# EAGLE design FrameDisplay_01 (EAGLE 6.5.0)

## Sheet 1 of 2: DISPLAY
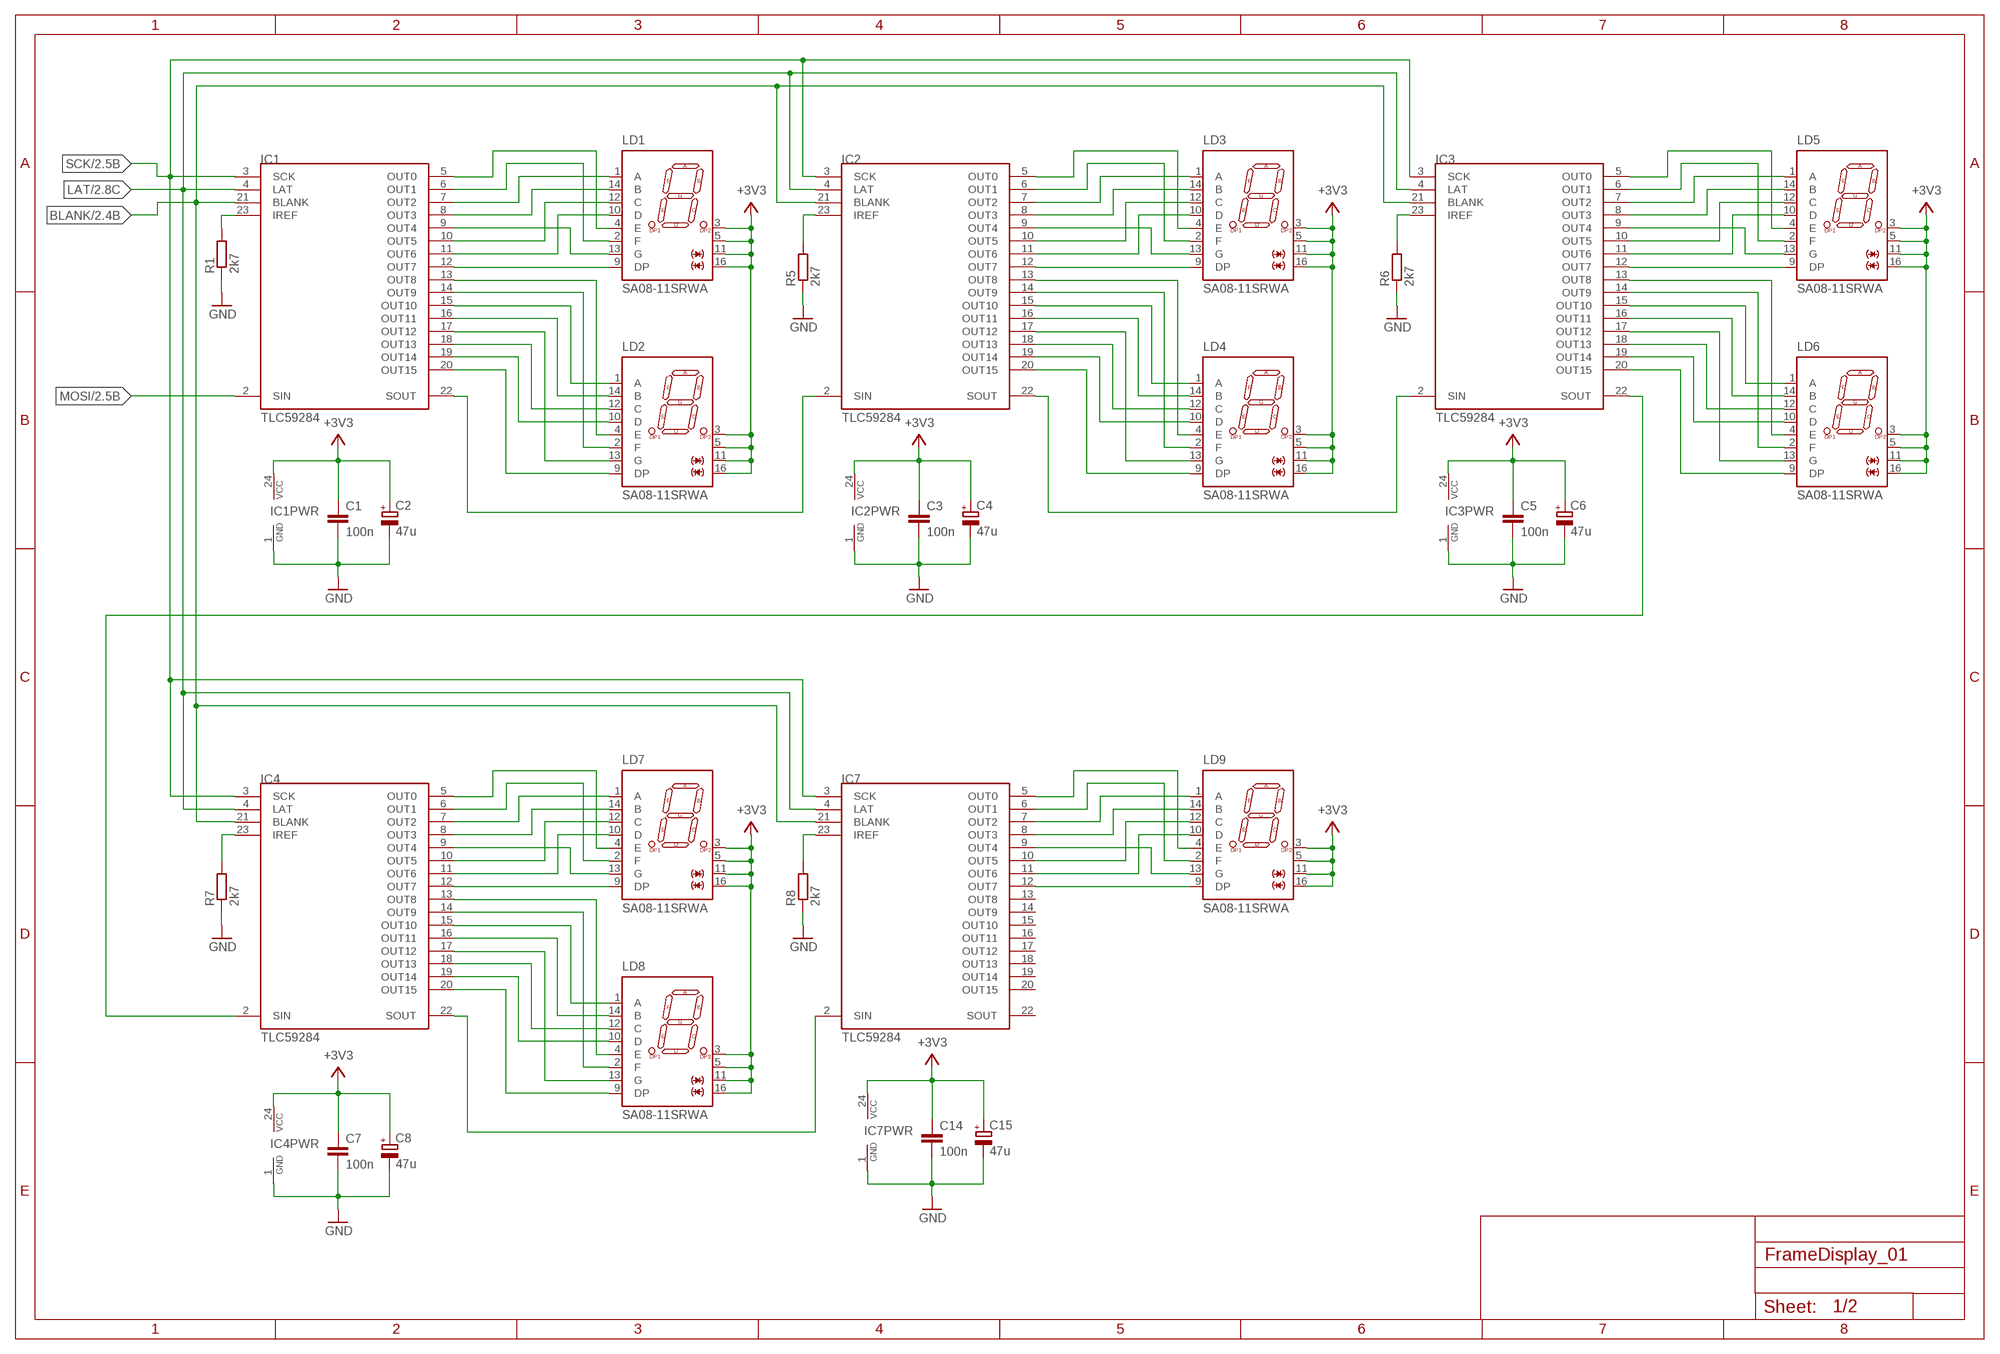
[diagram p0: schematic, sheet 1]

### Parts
C1  100n  C-EUC0603  [C0603]
C2  47u  CPOL-EUCT3216  [CT3216]
C3  100n  C-EUC0603  [C0603]
C4  47u  CPOL-EUCT3216  [CT3216]
C5  100n  C-EUC0603  [C0603]
C6  47u  CPOL-EUCT3216  [CT3216]
C7  100n  C-EUC0603  [C0603]
C8  47u  CPOL-EUCT3216  [CT3216]
C14  100n  C-EUC0603  [C0603]
C15  47u  CPOL-EUCT3216  [CT3216]
IC1  TLC59284  [SSOP24-25MIL]
IC2  TLC59284  [SSOP24-25MIL]
IC3  TLC59284  [SSOP24-25MIL]
IC4  TLC59284  [SSOP24-25MIL]
IC7  TLC59284  [SSOP24-25MIL]
LD1  SA08-11SRWA  SA08-11  [SA08]
LD2  SA08-11SRWA  SA08-11  [SA08]
LD3  SA08-11SRWA  SA08-11  [SA08]
LD4  SA08-11SRWA  SA08-11  [SA08]
LD5  SA08-11SRWA  SA08-11  [SA08]
LD6  SA08-11SRWA  SA08-11  [SA08]
LD7  SA08-11SRWA  SA08-11  [SA08]
LD8  SA08-11SRWA  SA08-11  [SA08]
LD9  SA08-11SRWA  SA08-11  [SA08]
R1  2k7  R-EU_R0603  [R0603]
R5  2k7  R-EU_R0603  [R0603]
R6  2k7  R-EU_R0603  [R0603]
R7  2k7  R-EU_R0603  [R0603]
R8  2k7  R-EU_R0603  [R0603]

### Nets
+3V3: C1.1 C2.+ C3.1 C4.+ C5.1 C6.+ C7.1 C8.+ C14.1 C15.+ IC1.24(PWR:VCC) IC2.24(PWR:VCC) IC3.24(PWR:VCC) IC4.24(PWR:VCC) IC7.24(PWR:VCC) LD1.3(AK) LD1.5(AK) LD1.11(AK) LD1.16(AK) LD2.3(AK) LD2.5(AK) LD2.11(AK) LD2.16(AK) LD3.3(AK) LD3.5(AK) LD3.11(AK) LD3.16(AK) LD4.3(AK) LD4.5(AK) LD4.11(AK) LD4.16(AK) LD5.3(AK) LD5.5(AK) LD5.11(AK) LD5.16(AK) LD6.3(AK) LD6.5(AK) LD6.11(AK) LD6.16(AK) LD7.3(AK) LD7.5(AK) LD7.11(AK) LD7.16(AK) LD8.3(AK) LD8.5(AK) LD8.11(AK) LD8.16(AK) LD9.3(AK) LD9.5(AK) LD9.11(AK) LD9.16(AK) ; also sheet 2
BLANK: IC1.21(BLANK) IC2.21(BLANK) IC3.21(BLANK) IC4.21(BLANK) IC7.21(BLANK) ; also sheet 2
GND: C1.2 C2.- C3.2 C4.- C5.2 C6.- C7.2 C8.- C14.2 C15.- IC1.1(PWR:GND) IC2.1(PWR:GND) IC3.1(PWR:GND) IC4.1(PWR:GND) IC7.1(PWR:GND) R1.1 R5.1 R6.1 R7.1 R8.1 ; also sheet 2
LAT: IC1.4(LAT) IC2.4(LAT) IC3.4(LAT) IC4.4(LAT) IC7.4(LAT) ; also sheet 2
MOSI: IC1.2(SIN) ; also sheet 2
N$1: IC1.12(OUT7) LD1.9(DP)
N$2: IC1.11(OUT6) LD1.10(D)
N$3: IC1.10(OUT5) LD1.12(C)
N$4: IC1.9(OUT4) LD1.13(G)
N$5: IC1.8(OUT3) LD1.14(B)
N$6: IC1.7(OUT2) LD1.1(A)
N$7: IC1.6(OUT1) LD1.2(F)
N$8: IC1.5(OUT0) LD1.4(E)
N$9: IC1.13(OUT8) LD2.4(E)
N$10: IC1.14(OUT9) LD2.2(F)
N$11: IC1.15(OUT10) LD2.1(A)
N$12: IC1.16(OUT11) LD2.14(B)
N$13: IC1.17(OUT12) LD2.13(G)
N$14: IC1.18(OUT13) LD2.12(C)
N$15: IC1.19(OUT14) LD2.10(D)
N$16: IC1.20(OUT15) LD2.9(DP)
N$17: IC4.12(OUT7) LD7.9(DP)
N$21: IC2.12(OUT7) LD3.9(DP)
N$22: IC2.11(OUT6) LD3.10(D)
N$23: IC2.10(OUT5) LD3.12(C)
N$24: IC2.9(OUT4) LD3.13(G)
N$25: IC2.8(OUT3) LD3.14(B)
N$26: IC2.7(OUT2) LD3.1(A)
N$27: IC2.6(OUT1) LD3.2(F)
N$28: IC2.5(OUT0) LD3.4(E)
N$29: IC2.13(OUT8) LD4.4(E)
N$30: IC2.14(OUT9) LD4.2(F)
N$31: IC2.15(OUT10) LD4.1(A)
N$32: IC2.16(OUT11) LD4.14(B)
N$33: IC2.17(OUT12) LD4.13(G)
N$34: IC2.18(OUT13) LD4.12(C)
N$35: IC2.19(OUT14) LD4.10(D)
N$36: IC2.20(OUT15) LD4.9(DP)
N$39: IC3.12(OUT7) LD5.9(DP)
N$40: IC3.11(OUT6) LD5.10(D)
N$41: IC3.10(OUT5) LD5.12(C)
N$42: IC3.9(OUT4) LD5.13(G)
N$43: IC3.8(OUT3) LD5.14(B)
N$44: IC3.7(OUT2) LD5.1(A)
N$45: IC3.6(OUT1) LD5.2(F)
N$46: IC3.5(OUT0) LD5.4(E)
N$47: IC3.13(OUT8) LD6.4(E)
N$48: IC3.14(OUT9) LD6.2(F)
N$49: IC3.15(OUT10) LD6.1(A)
N$50: IC3.16(OUT11) LD6.14(B)
N$51: IC3.17(OUT12) LD6.13(G)
N$52: IC3.18(OUT13) LD6.12(C)
N$53: IC3.19(OUT14) LD6.10(D)
N$54: IC3.20(OUT15) LD6.9(DP)
N$57: IC4.11(OUT6) LD7.10(D)
N$58: IC4.10(OUT5) LD7.12(C)
N$59: IC4.9(OUT4) LD7.13(G)
N$60: IC4.8(OUT3) LD7.14(B)
N$61: IC4.7(OUT2) LD7.1(A)
N$62: IC4.6(OUT1) LD7.2(F)
N$63: IC4.5(OUT0) LD7.4(E)
N$64: IC4.13(OUT8) LD8.4(E)
N$65: IC4.14(OUT9) LD8.2(F)
N$66: IC4.15(OUT10) LD8.1(A)
N$67: IC4.16(OUT11) LD8.14(B)
N$68: IC4.17(OUT12) LD8.13(G)
N$69: IC4.18(OUT13) LD8.12(C)
N$70: IC4.19(OUT14) LD8.10(D)
N$71: IC4.20(OUT15) LD8.9(DP)
N$72: IC1.22(SOUT) IC2.2(SIN)
N$73: IC2.22(SOUT) IC3.2(SIN)
N$74: IC3.22(SOUT) IC4.2(SIN)
N$75: IC4.22(SOUT) IC7.2(SIN)
N$76: IC1.23(IREF) R1.2
N$77: IC2.23(IREF) R5.2
N$78: IC3.23(IREF) R6.2
N$79: IC4.23(IREF) R7.2
N$80: IC7.23(IREF) R8.2
N$88: IC7.12(OUT7) LD9.9(DP)
N$89: IC7.11(OUT6) LD9.10(D)
N$90: IC7.10(OUT5) LD9.12(C)
N$91: IC7.9(OUT4) LD9.13(G)
N$92: IC7.8(OUT3) LD9.14(B)
N$93: IC7.7(OUT2) LD9.1(A)
N$94: IC7.6(OUT1) LD9.2(F)
N$95: IC7.5(OUT0) LD9.4(E)
SCK: IC1.3(SCK) IC2.3(SCK) IC3.3(SCK) IC4.3(SCK) IC7.3(SCK) ; also sheet 2
Unconnected: IC7.13(OUT8) IC7.14(OUT9) IC7.15(OUT10) IC7.16(OUT11) IC7.17(OUT12) IC7.18(OUT13) IC7.19(OUT14) IC7.20(OUT15) IC7.22(SOUT)

## Sheet 2 of 2: CPU
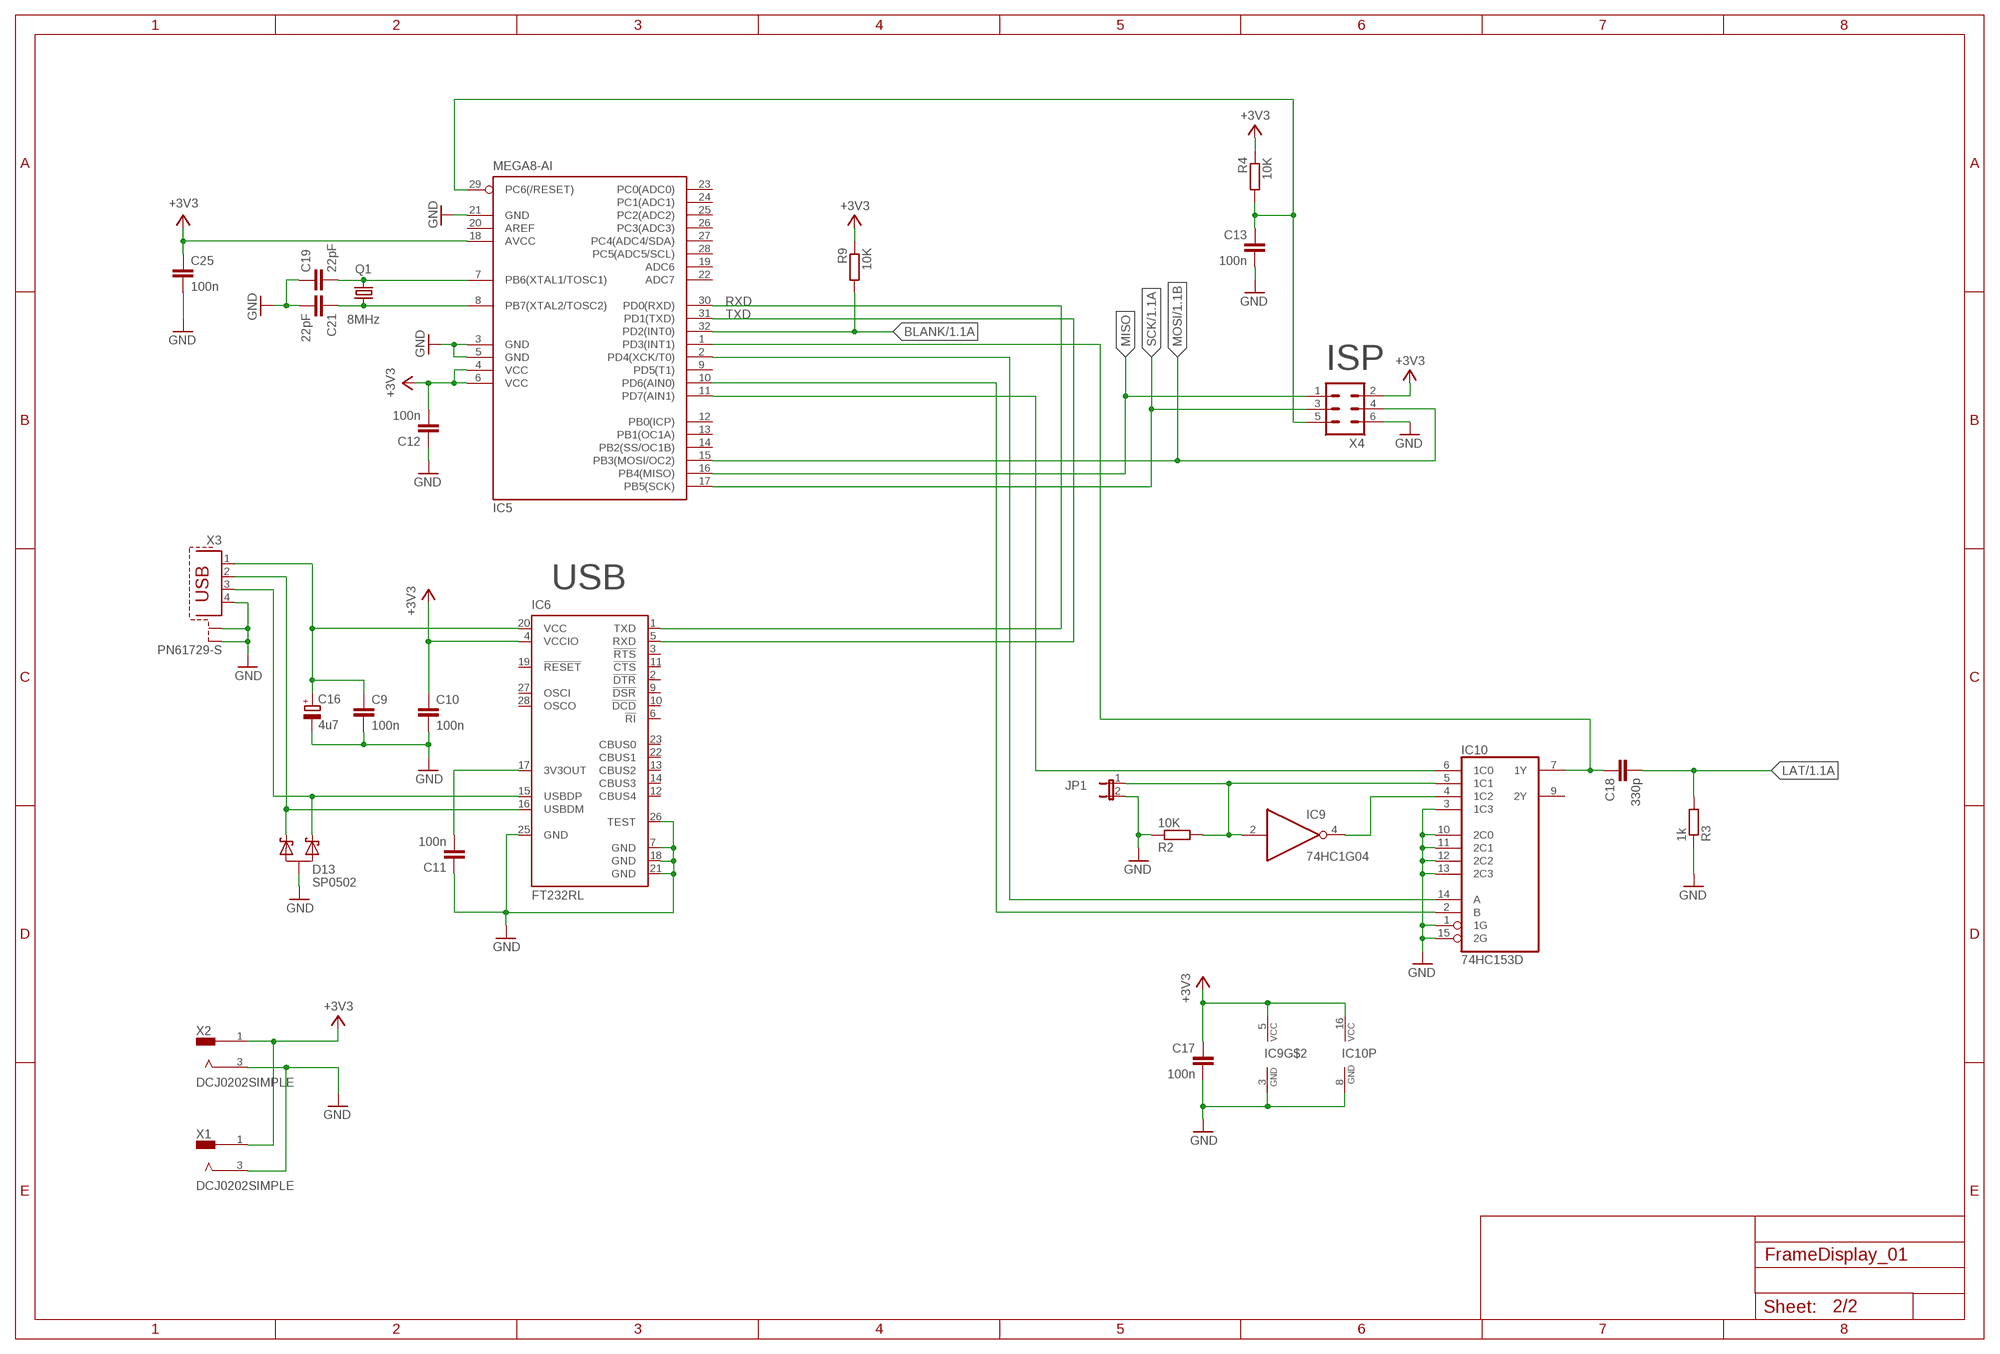
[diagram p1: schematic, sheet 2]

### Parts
C9  100n  C-EUC0603  [C0603]
C10  100n  C-EUC0603  [C0603]
C11  100n  C-EUC0603  [C0603]
C12  100n  C-EUC0603  [C0603]
C13  100n  C-EUC0603  [C0603]
C16  4u7  CPOL-EUSMCA  [SMC_A]
C17  100n  C-EUC0603  [C0603]
C18  330p  C-EUC0603  [C0603]
C19  22pF  C-EUC0603  [C0603]
C21  22pF  C-EUC0603  [C0603]
C25  100n  C-EUC0603  [C0603]
D13  SP0502  [SOT23]
IC5  MEGA8-AI  [TQFP32-08]
IC6  FT232RL  [SSOP28]
IC9  74HC1G04  74AHC1GU04DBV  [SOT23-5]
IC10  74HC153D  74HCT153D  [SO16]
JP1  JP1E  [JP1]
Q1  8MHz  CRYSTALCTS406  [CTS406]
R2  10K  R-EU_R0603  [R0603]
R3  1k  R-EU_R0603  [R0603]
R4  10K  R-EU_R0603  [R0603]
R9  10K  R-EU_R0603  [R0603]
X1  DCJ0202SIMPLE  [DCJ0202_SIMPLE]
X2  DCJ0202SIMPLE  [DCJ0202_SIMPLE]
X3  PN61729-S  [PN61729-S]
X4  ML6  [ML6]

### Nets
+3V3: C10.1 C12.2 C17.1 C25.1 IC5.4(VCC) IC5.6(VCC) IC5.18(AVCC) IC6.4(VCCIO) IC9.5(VCC) IC10.16(VCC) R4.1 R9.1 X1.1 X2.1 X4.2 ; also sheet 1
BLANK: IC5.32(PD2(INT0)) R9.2 ; also sheet 1
GND: C9.2 C10.2 C11.1 C12.1 C13.2 C16.- C17.2 C19.1 C21.2 C25.2 D13.3(GND) IC5.3(GND) IC5.5(GND) IC5.21(GND) IC6.7(GND) IC6.18(GND) IC6.21(GND) IC6.25(GND) IC6.26(TEST) IC9.3(GND) IC10.1(1G) IC10.3(1C3) IC10.8(GND) IC10.10(2C0) IC10.11(2C1) IC10.12(2C2) IC10.13(2C3) IC10.15(2G) JP1.2 R2.1 R3.1 X1.3 X2.3 X3.4 X3.S1 X3.S2 X4.6 ; also sheet 1
LAT: C18.2 R3.2 ; also sheet 1
LAT_CPU: IC5.11(PD7(AIN1)) IC10.6(1C0)
LAT_IN: C18.1 IC5.1(PD3(INT1)) IC10.7(1Y)
MISO: IC5.16(PB4(MISO)) X4.1
MOSI: IC5.15(PB3(MOSI/OC2)) X4.4 ; also sheet 1
N$19: C9.1 C16.+ IC6.20(VCC) X3.1
N$20: D13.2(C0) IC6.16(USBDM) X3.2
N$37: D13.1(C1) IC6.15(USBDP) X3.3
N$38: C21.1 IC5.8(PB7(XTAL2/TOSC2)) Q1.1
N$55: C19.2 IC5.7(PB6(XTAL1/TOSC1)) Q1.3
N$81: IC5.2(PD4(XCK/T0)) IC10.14(A)
N$82: IC5.10(PD6(AIN0)) IC10.2(B)
N$85: IC9.4(O) IC10.4(1C2)
N$86: C11.2 IC6.17(3V3OUT)
RESET: C13.1 IC5.29(PC6(/RESET)) R4.2 X4.5
RXD: IC5.30(PD0(RXD)) IC6.1(TXD)
SCK: IC5.17(PB5(SCK)) X4.3 ; also sheet 1
SYNC: IC9.2(I) IC10.5(1C1) JP1.1 R2.2
TXD: IC5.31(PD1(TXD)) IC6.5(RXD)
Unconnected: IC5.9(PD5(T1)) IC5.12(PB0(ICP)) IC5.13(PB1(OC1A)) IC5.14(PB2(SS/OC1B)) IC5.19(ADC6) IC5.20(AREF) IC5.22(ADC7) IC5.23(PC0(ADC0)) IC5.24(PC1(ADC1)) IC5.25(PC2(ADC2)) IC5.26(PC3(ADC3)) IC5.27(PC4(ADC4/SDA)) IC5.28(PC5(ADC5/SCL)) IC6.2(!DTR) IC6.3(!RTS) IC6.6(!RI) IC6.9(!DSR) IC6.10(!DCD) IC6.11(!CTS) IC6.12(CBUS4) IC6.13(CBUS2) IC6.14(CBUS3) IC6.19(!RESET) IC6.22(CBUS1) IC6.23(CBUS0) IC6.27(OSCI) IC6.28(OSCO) IC10.9(2Y)

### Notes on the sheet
- ISP
- USB

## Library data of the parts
C1 C3 C5 C7 C9-C14 C17 C18 C25 = rcl:C-EU: CAPACITOR, European symbol
C2 C4 C6 C8 C15 = rcl:CPOL-EU: POLARIZED CAPACITOR, European symbol
C16 = rcl:CPOL-EU: POLARIZED CAPACITOR, European symbol; OC_FARNELL: unknown
C19 C21 = rcl:C-EU: CAPACITOR, European symbol; MF: AVX; MPN: 02013A220JAT2A; OC_FARNELL: 1327610
D13 = Brunner:SP0502; MF: LITTELFUSE; MPN: SP0502BAHTG; OC_FARNELL: 1827631
IC1-IC4 IC7 = Brunner:TLC59284
IC5 = atmel:MEGA8: MICROCONTROLLER 8 Kbytes FLASH, 1 kbytes SRAM, 512 bytes EEPROM, USART, 6-channel 10 bit ADC, 2-channel 8 bit ADC Pin compatible with Atmega48, ATMega88, ATMega168 Source: avr.lbr; MF: ATMEL; MPN: ATMEGA8-16AU; OC_FARNELL: 9171371; OC_NEWARK: 73M8863
IC6 = ftdichip:FT232R: Source: http://www.ftdichip.com/Documents/DataSheets/DS_FT232R_v104.pdf; MF: FTDI; MPN: FT232RL; OC_FARNELL: 1146032; OC_NEWARK: 91K9918
IC9 = 74xx-little-us:74*1GU04: Single Unbuffered Inverter
IC10 = 74xx-eu:74*153: Dual 4-line to 1-line data SELECTOR/MULTIPLEXER
JP1 = jumper:JP1E: JUMPER
LD1-LD9 = led:S*08: Kingbright 20mm (0.8Inch) Single Digit Numeric Display Source: SA08-11SRWA.pdf
Q1 = crystal:CRYSTAL: CRYSTAL; OC_FARNELL: unknown; OC_NEWARK: unknown
R1 R5-R8 = rcl:R-EU_: RESISTOR, European symbol
R2-R4 R9 = rcl:R-EU_: RESISTOR, European symbol; OC_FARNELL: unknown
X1 X2 = Brunner:DCJ0202: DC POWER JACK
X3 = con-berg:PN61729-S: BERG USB connector; OC_FARNELL: unknown; OC_NEWARK: unknown
X4 = con-ml:ML6: HARTING; OC_FARNELL: unknown; OC_NEWARK: unknown

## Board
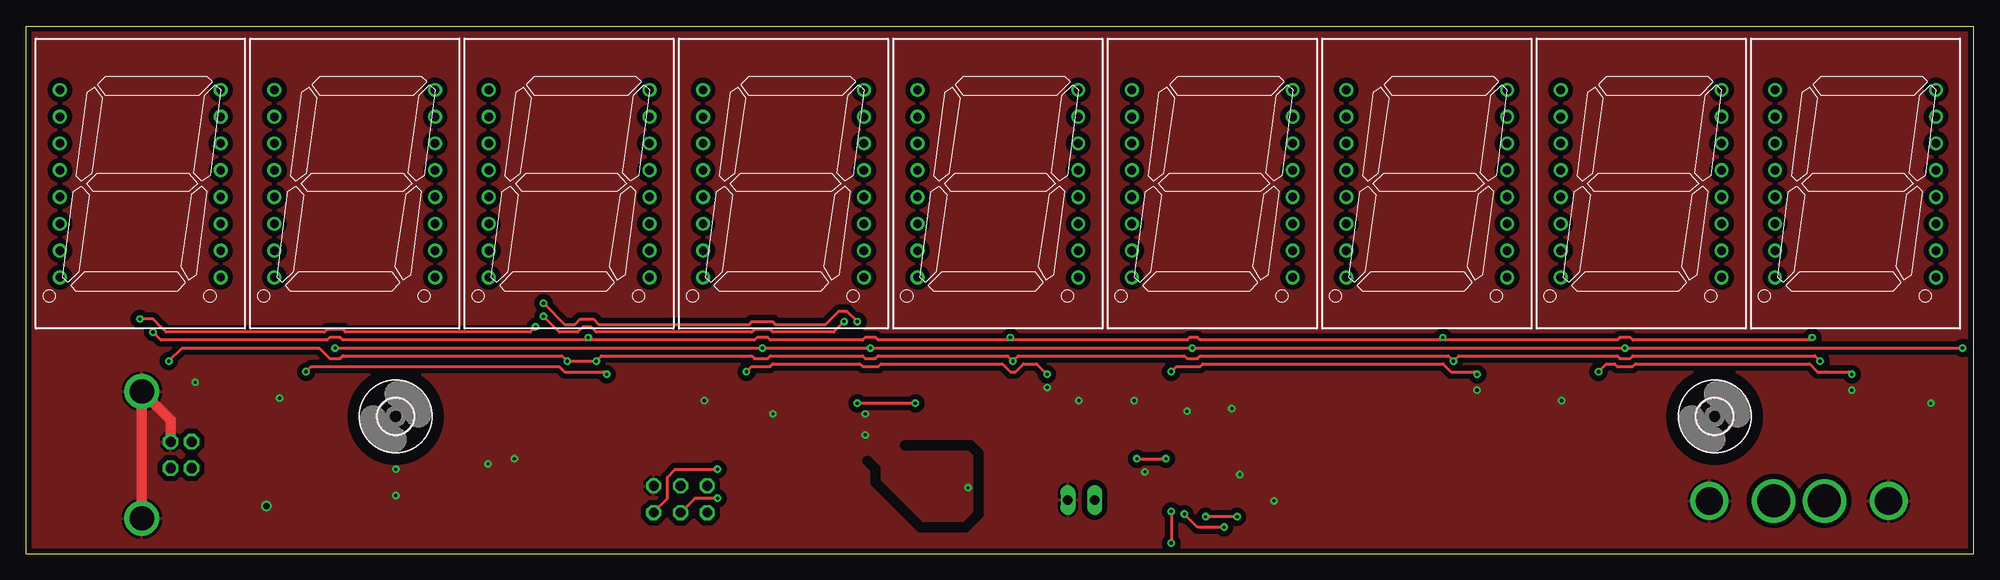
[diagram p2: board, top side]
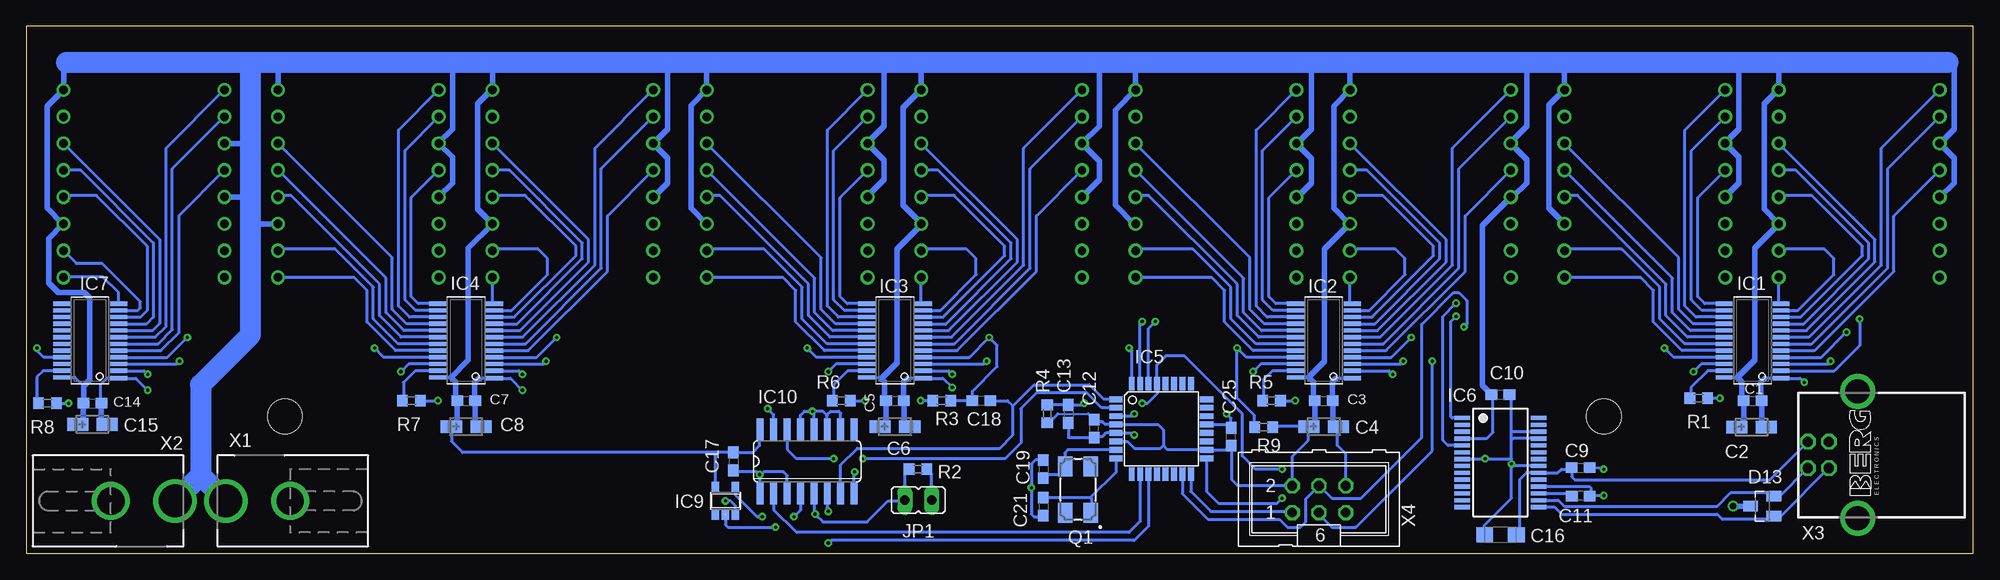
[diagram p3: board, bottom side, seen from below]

Size 184.5 x 50 mm. Coordinates in mm from the lower left corner, seen from the top.
Outline: 0,0 0,50 184.5,50 184.5,0 0,0
Copper layers (1*16): Top 0.035mm / dielectric 1.5mm / Bottom 0.035mm
Design rules "default *": minimum track width 0.2mm, minimum drill 0.3mm, track to track 0.3mm, track to pad 0.25mm, pad to pad 0.23mm, via to via 0.3mm, smd to smd 0.2mm, copper to edge 0.5mm, drill to drill 0.2mm, minimum pad ring 10mil, minimum via ring 8mil, stop-mask expansion 4mil, vias tented up to drill 0.5mm, thermal gap 10mil
tRestrict: 8 lines

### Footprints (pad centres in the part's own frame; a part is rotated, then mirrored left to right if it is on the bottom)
C0603 = smd 1.1 x 1: 1 -0.85,0; 2 0.85,0
CT3216 = smd 2 x 1.2: + -1.4,0; - 1.4,0
SMC_A = smd 1.6 x 1.4: + -1.5,0; - 1.5,0
SOT23 = smd 1 x 1.4: 1 -0.95,-1.1; 2 0.95,-1.1; 3 0,1.1
SSOP24-25MIL = smd 0.4 x 1.6: 1 -3.575,-2.7; 2 -2.857,-2.7; 3 -2.223,-2.7; 4 -1.587,-2.7; 5 -0.953,-2.7; 6 -0.318,-2.7; 7 0.318,-2.7; 8 0.953,-2.7; 9 1.587,-2.7; 10 2.223,-2.7; 11 2.857,-2.7; 12 3.493,-2.7; 13 3.493,2.7; 14 2.857,2.7; 15 2.223,2.7; 16 1.587,2.7; 17 0.953,2.7; 18 0.318,2.7; 19 -0.318,2.7; 20 -0.953,2.7; 21 -1.587,2.7; 22 -2.223,2.7; 23 -2.857,2.7; 24 -3.493,2.7
TQFP32-08 = smd 1.27 x 0.559: 1 -4.293,2.8; 2 -4.293,2; 3 -4.293,1.2; 4 -4.293,0.4; 5 -4.293,-0.4; 6 -4.293,-1.2; 7 -4.293,-2; 8 -4.293,-2.8; 17 4.293,-2.8; 18 4.293,-2; 19 4.293,-1.2; 20 4.293,-0.4; 21 4.293,0.4; 22 4.293,1.2; 23 4.293,2; 24 4.293,2.8 | smd 0.559 x 1.27: 9 -2.8,-4.293; 10 -2,-4.293; 11 -1.2,-4.293; 12 -0.4,-4.293; 13 0.4,-4.293; 14 1.2,-4.293; 15 2,-4.293; 16 2.8,-4.293; 25 2.8,4.293; 26 2,4.293; 27 1.2,4.293; 28 0.4,4.293; 29 -0.4,4.293; 30 -1.2,4.293; 31 -2,4.293; 32 -2.8,4.293
SSOP28 = smd 0.4 x 1.5: 1 -4.225,-3.625; 2 -3.575,-3.625; 3 -2.925,-3.625; 4 -2.275,-3.625; 5 -1.625,-3.625; 6 -0.975,-3.625; 7 -0.325,-3.625; 8 0.325,-3.625; 9 0.975,-3.625; 10 1.625,-3.625; 11 2.275,-3.625; 12 2.925,-3.625; 13 3.575,-3.625; 14 4.225,-3.625; 15 4.225,3.625; 16 3.575,3.625; 17 2.925,3.625; 18 2.275,3.625; 19 1.625,3.625; 20 0.975,3.625; 21 0.325,3.625; 22 -0.325,3.625; 23 -0.975,3.625; 24 -1.625,3.625; 25 -2.275,3.625; 26 -2.925,3.625; 27 -3.575,3.625; 28 -4.225,3.625
SOT23-5 = smd 0.69 x 0.99: 1 -0.95,-1.29; 2 0,-1.29; 3 0.95,-1.29; 4 0.95,1.3; 5 -0.95,1.3
SO16 = smd 0.66 x 2.032: 1 -4.445,-3.073; 2 -3.175,-3.073; 3 -1.905,-3.073; 4 -0.635,-3.073; 5 0.635,-3.073; 6 1.905,-3.073; 7 3.175,-3.073; 8 4.445,-3.073; 9 4.445,3.073; 10 3.175,3.073; 11 1.905,3.073; 12 0.635,3.073; 13 -0.635,3.073; 14 -1.905,3.073; 15 -3.175,3.073; 16 -4.445,3.073
JP1 = drill 0.914 long: 1 0,-1.27; 2 0,1.27
SA08 = drill 0.8 pad 1.27: 1 -7.62,8.89; 2 -7.62,6.35; 3 -7.62,3.81; 4 -7.62,1.27; 5 -7.62,-1.27; 6 -7.62,-3.81; 7 -7.62,-6.35; 8 -7.62,-8.89; 9 7.62,-8.89; 10 7.62,-6.35; 11 7.62,-3.81; 12 7.62,-1.27; 13 7.62,1.27; 14 7.62,3.81; 15 7.62,6.35; 16 7.62,8.89
CTS406 = smd 1.9 x 1.4: 1 -2.2,-1.2; 2 2.2,-1.2; 3 2.2,1.2; 4 -2.2,1.2
R0603 = smd 1 x 1.1: 1 -0.85,0; 2 0.85,0
3,3 = hole 3.3: 0,0
DCJ0202_SIMPLE = drill 3.1: 1 0,3.1 | drill 2.6: 3 0,-3
PN61729-S = drill 0.95 octagon: 1 1.25,4.71; 2 -1.25,4.71; 3 -1.25,2.71; 4 1.25,2.71 | drill 2.3 pad 2.9: S1 -6.02,0; S2 6.02,0
ML6 = drill 0.914 octagon: 1 -2.54,-1.27; 2 -2.54,1.27; 3 0,-1.27; 4 0,1.27; 5 2.54,-1.27; 6 2.54,1.27

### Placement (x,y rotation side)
C1  20.9,14.49 0 bottom
C2  21,12 0 bottom
C3  61.54,14.49 0 bottom
C4  61.54,12.04 0 bottom
C5  102.18,14.49 0 bottom
C6  102.18,12.04 0 bottom
C7  142.82,14.49 0 bottom
C8  142.82,12.04 0 bottom
C9  37.2,8.14 0 bottom
C10  44.8,15.09 0 bottom
C11  37.18,5.46 180 bottom
C12  83.29,11.84 90 bottom
C13  85.75,13.25 270 bottom
C14  178.25,14.25 0 bottom
C15  178.25,12.25 0 bottom
C16  44.8,1.78 180 bottom
C17  117.5,8.75 270 bottom
C18  94,14.5 180 bottom
C19  88.12,8.03 270 bottom
C21  88.12,4.47 270 bottom
C25  70.34,11.08 90 bottom
D13  20,4.5 90 bottom
IC1  20.9,20.2 90 bottom
IC2  61.54,20.2 90 bottom
IC3  102.18,20.2 90 bottom
IC4  142.82,20.2 90 bottom
IC5  76.94,11.84 0 bottom
IC6  44.8,8.64 270 bottom
IC7  178.46,20.2 90 bottom
IC9  118.25,5 0 bottom
IC10  110.5,8.75 0 bottom
JP1  99.97,5.08 270 bottom
LD1  10.79,35.09 0 top
LD2  31.11,35.09 0 top
LD3  51.44,35.09 0 top
LD4  71.75,35.09 0 top
LD5  92.08,35.09 0 top
LD6  112.39,35.09 0 top
LD7  132.72,35.09 0 top
LD8  153.03,35.09 0 top
LD9  173.35,35.09 0 top
Q1  84.84,6.09 90 bottom
R1  26,14.75 180 bottom
R2  100,8 180 bottom
R3  97.75,14.5 0 bottom
R4  87.75,13.25 90 bottom
R5  66.5,14.5 180 bottom
R6  107.25,14.5 180 bottom
R7  148,14.5 180 bottom
R8  182.5,14.25 180 bottom
R9  67.25,12 180 bottom
U$1  [3,3]  35,13 0 top
U$2  [3,3]  160,13 0 top
X1  162.5,5 90 bottom
X2  173.5,5 270 bottom
X3  10.95,9.36 90 bottom
X4  61.99,5.16 0 bottom

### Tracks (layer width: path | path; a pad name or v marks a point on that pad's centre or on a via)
+3V3
  Bottom 0.2: 86.75,13.25 83.85,13.25
  Bottom 0.3: LD7.5 125.06,33.81 | LD7.16 140.41,43.98 | 1.8,45.96 2.4,46.56 | 42.3,46.26 42,46.56 | 38.73,46.52 38.7,46.56 | 18.41,46.45 18.3,46.56 | 59.05,46.3 58.8,46.56 | 79.38,46.44 79.5,46.56 | 99.69,46.47 99.6,46.56 | 160.66,46.52 160.62,46.56 | 140.34,46.45 140.22,46.56 | 180.97,46.3 180.72,46.56 | 123.72,46.44 123.6,46.56 | IC7.24 179.91,16.71 179.09,15.88 | 181.06,31.25 181.03,31.25 181.03,31.27 LD9.11 | IC4.24 144.27,16.71 | IC1.24 22.35,16.71 | IC2.24 62.99,16.71 | 59.12,31.25 59.12,31.27 LD3.11 | IC3.24 103.63,16.71 103.49,16.57 | LD5.5 | 99.69,31.36 LD5.11 99.69,31.16 | LD3.5 43.65,33.81 | LD1.5 3.15,33.81 | LD1.16 18.48,43.98 | LD2.5 23.5,33.87 | LD2.11 38.73,31.3 | LD4.5 64.05,33.81 | LD4.11 79.52,31.27 | LD6.5 104.78,33.88 | LD6.16 | LD8.5 145.41,33.87 | LD3.3 43.81,39.05 | LD2.3 23.5,38.97 | LD1.3 | LD4.3 64.06,38.9 | LD5.3 | LD6.3 104.78,38.98 | 120.02,46.55 120,46.56 | LD7.3 | LD8.3 145.41,38.97 | 86.75,13.25 87.6,12.4 R4.1 | 83.85,13.25 C12.2 83.1,12.5 82.5,12.5 82.24,12.24 IC5.4 77.24,12.24 76.75,11.75 76.75,10.25 | IC5.6 80.14,10.64 79.5,10 77,10 76.75,10.25 | 76.75,10.25 76.34,9.84 IC5.18 70.72,9.84 C25.1 70.25,10.14 70.25,7 69.68,6.43 X4.2 64.53,9.22 63,10.75 63,11.98 C4.+ 66.36,12.04 R9.1 | IC6.4 46.09,10.91 45.5,11.5 45.5,14.93 C10.1 | IC10.16 115,11.77 115,10.25 115.65,9.6 C17.1 119,9.6 | 119,9.6 143.16,9.6 144.22,10.66 C8.+ | 163.35,38.9 163.25,39 | 163.31,33.81 163.25,33.75 | 163.03,31.27 163.25,31.5 | IC9.5 119.2,9.4 119,9.6
  Bottom 0.305: IC5.6 80.31,10.64
  Bottom 0.5: 125.06,33.81 123.72,35.16 123.72,37.52 LD7.3 | 140.41,43.98 141.72,42.66 141.72,32.66 LD7.11 142.62,28.99 142.62,18.36 144.27,16.71 | LD1.3 1.8,40.26 1.8,45.96 | 23.5,38.97 22.2,40.26 22.2,46.56 | 43.81,39.05 42.3,40.56 42.3,46.26 | 64.06,38.9 62.7,40.26 62.7,46.56 | LD5.3 82.8,40.56 82.8,46.56 | 104.78,38.98 103.2,40.56 103.2,46.56 | LD7.3 123.72,40.26 123.72,46.44 | 145.41,38.97 144.12,40.26 144.12,46.56 | 180.97,46.3 LD9.16 182.52,42.43 182.52,32.76 181.03,31.27 | 181.06,31.25 182.4,29.9 182.4,25.65 181.5,24.75 179,24.75 178.5,24.25 178.5,16.47 179.09,15.88 179.09,14.27 C14.1 179.1,12.6 179,12.5 179.4,12.5 C15.+ | 144.27,16.71 143.82,16.26 143.82,14.62 143.79,14.62 C7.1 143.67,12.6 C8.+ | 22.35,16.71 21.9,16.26 21.9,14.62 21.88,14.62 C1.1 21.75,12.65 C2.+ | 22.35,16.71 20.7,18.36 20.7,28.99 LD1.11 19.8,32.66 19.8,42.66 18.48,43.98 | 59.12,31.27 60.6,32.76 60.6,42.43 LD3.16 59.05,46.3 | 59.12,31.25 61.5,28.86 61.5,18.2 62.99,16.71 62.54,16.26 62.54,14.62 62.52,14.62 C3.1 62.39,12.6 C4.+ | 99.69,31.16 102,28.86 102,18.06 103.49,16.57 103.18,16.26 103.18,14.62 103.16,14.62 C5.1 103.03,12.6 C6.+ | LD5.5 82.8,35.46 82.8,37.24 LD5.3 | 99.69,31.36 101.4,33.06 101.4,42.27 LD5.16 99.69,46.47 | 43.65,33.81 42.3,35.16 42.3,37.38 LD3.3 | LD3.5 46.5,31.13 46.5,15.93 C10.1 | 3.15,33.81 1.8,35.16 1.8,37.52 LD1.3 | 23.5,33.87 22.2,35.16 22.2,37.6 LD2.3 | 38.73,31.3 40.2,32.76 40.2,42.51 LD2.16 38.73,46.52 | 64.05,33.81 62.7,35.16 62.7,37.46 LD4.3 | 79.52,31.27 81.3,33.06 81.3,42.05 LD4.16 79.38,46.44 | 104.78,33.88 103.2,35.46 103.2,37.32 LD6.3 | LD6.16 121.5,42.5 121.5,32.76 LD6.11
  Bottom 0.5: 145.41,33.87 144.12,35.16 144.12,37.6 LD8.3 | LD1.16 18.41,46.45 | LD6.16 120.02,46.55 | LD7.16 140.34,46.45 | LD8.16 160.66,46.52 | LD9.3 163.35,38.9 | LD9.5 163.31,33.81 | LD8.11 163.03,31.27
  Bottom 1: 163.25,46.56 163,46.56
  Bottom 2: 2.4,46.56 18.3,46.56 22.2,46.56 38.7,46.56 42,46.56 58.8,46.56 62.7,46.56 79.5,46.56 82.8,46.56 99.6,46.56 103.2,46.56 120,46.56 123.6,46.56 140.22,46.56 144.12,46.56 160.62,46.56 163,46.56 | 180.72,46.56 163.25,46.56 163.25,39 163.25,33.75 163.25,31.5 163.25,20.75 168,16 168,7.4 | 168,7.4 X1.1 | X2.1 168,7.4
BLANK  (via drill 0.3)
  Top 0.3: v29.25,19.5 v69.75,19.5 v80,19.5 v110.5,19.5 v151.5,19.5 v183.5,19.5
  Bottom 0.3: IC1.21 28.37,18.62 v29.25,19.5 | IC2.21 68.87,18.62 v69.75,19.5 69.75,14.75 68.1,13.1 R9.2 | IC3.21 109.62,18.62 v110.5,19.5 | IC4.21 150.62,18.62 v151.5,19.5 | IC7.21 182.87,18.62 183.5,19.25 v183.5,19.5 | IC5.32 79.74,19.24 v80,19.5
GND  (via drill 0.3, 0.6)
  Top 1: X3.4 13.66,12.67 X3.S2 X3.S1
  Bottom 0.25: C9.2 35.14,8.14 v35,8
  Bottom 0.3: 19.73,16.63 IC1.1 16.38,16.63 v16,16.25 | IC2.1 60.37,16.63 | 101.01,16.63 IC3.1 97.63,16.63 v96.75,15.75 | 141.65,16.63 IC4.1 138.63,16.63 v137.5,15.5 | IC5.5 79.69,11.44 v79.5,11.25 | C12.1 85.75,10.99 C13.2 | 88,9 C19.1 88.87,8.88 89.25,8.5 v89.25,6.25 89.25,3.75 89,3.5 88.24,3.5 C21.2 | IC10.8 106.06,7.7 v106,7.75 | IC10.15 113.67,13.18 v114.25,13.75 | IC10.13 111.14,13.12 110.75,13.5 v110,13.5 | JP1.2 98.7,7.55 R2.1 | IC6.18 36.37,6.37 36.25,6.25 36.25,5.54 | 36.25,5.54 C11.1 | 36.25,5.54 35.05,5.54 v35,5.5 | X4.6 59.45,9.45 60.25,10.25 60.25,11.94 C4.- | R5.1 v64.25,14.5 | C25.2 70.34,12.84 v70.75,13.25 | IC5.3 79.71,13.04 v79.5,13.25 | R6.1 v105,14.5 | R7.1 v145.5,14.5 | R1.1 v24,14.75 | C16.- 46.3,2.7 43.75,5.25 v43.75,8.5 | v43.75,8.5 43.75,9 | 43.75,9 43.75,10.75 | 43.75,10.75 43.75,11.5 | 43.75,11.5 43.75,14.88 C10.2 | IC6.7 46.28,8.96 v46.25,9 43.75,9 | IC6.21 43.56,8.31 v43.75,8.5 | IC6.26 43.69,11.56 43.75,11.5 | IC6.25 43.59,10.91 43.75,10.75 | v173,15.5 174.13,16.63 IC7.1 176.87,16.63 177.5,16 177.5,14.4 | R8.1 v180.5,14.25 | v110,13.5 109,13.5 108.59,13.1 IC10.11 108.59,13.15 108.25,13.5 107.5,13.5 107.33,13.32 IC10.10 | IC10.12 109.86,13.37 v110,13.5 | IC9.3 117.3,4.55 117.75,5 v118.25,5 | IC10.1 114.94,7.45 | 114.94,7.45 v115,7.5 115.25,7.75 117.35,7.75 C17.2 | IC10.3 112.41,7.41 112.75,7.75 114.64,7.75 114.94,7.45 | R3.1 v99.75,14.5
  Bottom 0.305: IC5.21 70.65,12.24 C25.2 | IC5.5 82.17,11.44 82.53,11.08 83.2,11.08 C12.1
  Bottom 0.5: 19.73,16.63 20.1,16.26 20.1,14.54 C1.2 20.05,12.45 C2.- | 60.37,16.63 60.74,16.26 60.74,14.54 C3.2 60.69,12.6 C4.- | 101.01,16.63 101.38,16.26 101.38,14.54 C5.2 101.33,12.6 C6.- | 141.65,16.63 142.02,16.26 142.02,14.54 C7.2 141.97,12.6 C8.- | D13.3 v22.75,4.5 | C15.- 177.1,12.5 177.25,12.5 177.4,12.65 C14.2 177.5,14.35 177.5,14.4
  pour Top (isolate 0.5): 0,0 0,50 185,50 185,0
LAT  (via drill 0.3)
  Top 0.3: v169.25,20.5 169,20.25 152.25,20.25 152,20.5 151,20.5 150.75,20.25 134.5,20.25 v134.25,20.5 134,20.25 111.25,20.25 111,20.5 110.25,20.5 110,20.25 93.5,20.25 v93.25,20.5 93,20.25 80.75,20.25 80.5,20.5 79.5,20.5 79.25,20.25 70.5,20.25 70.25,20.5 69.25,20.5 69,20.25 53.5,20.25 v53.25,20.5 53,20.25 30,20.25 29.75,20.5 28.75,20.5 28.5,20.25 12.75,20.25 v12,21
  Bottom 0.3: IC7.4 171.13,18.62 v169.25,20.5 | IC1.4 14.38,18.62 v12,21 | IC2.4 55.13,18.62 v53.25,20.5 | IC4.4 136.13,18.62 v134.25,20.5 | IC3.4 95.13,18.62 v93.25,20.5 92.5,19.75 92.5,17.75 94.85,15.4 C18.2 R3.2
LAT_CPU  (via drill 0.3)
  Top 0.3: v108.5,4 v108.5,1
  Bottom 0.3: IC5.11 78.14,2.61 79.5,1.25 108.25,1.25 v108.5,1 | IC10.6 108.59,4.09 v108.5,4
LAT_IN
  Bottom 0.3: IC10.7 107.33,8.43 105.75,10 92.25,10 91,11.25 91,14 | 91,14 89,16 83.75,16 82.39,14.64 IC5.1 | C18.1 91.5,14.5 91,14
MISO
  Bottom 0.3: IC5.16 74.14,5.89 72.25,4 64.64,4 X4.1
MOSI  (via drill 0.3)
  Top 0.3: v48.25,21.5 48,21.25 47.75,21 30.25,21 30,21.25 28.5,21.25 28.25,21 13.25,21 12.75,21.5 12,22.25 v10.75,22.25
  Bottom 0.3: IC5.15 74.94,5.69 72.5,3.25 65.75,3.25 65,2.5 63.75,2.5 63.25,3 63.25,5.17 X4.4 61.93,6.43 60.75,5.25 58,5.25 52.25,11 52.25,21.75 49.25,24.75 48.75,24.75 48,24 48,21.75 v48.25,21.5 | v10.75,22.25 10.75,19.75 13.15,17.35 IC1.2
N$1
  Bottom 0.3: IC1.12 18.41,23.7 LD1.9
N$2
  Bottom 0.3: IC1.11 16.6,23.06 13.2,26.46 13.2,27.96 14.1,28.86 18.29,28.86 LD1.10
N$3
  Bottom 0.3: IC1.10 16.33,22.43 10.5,28.26 10.5,29.16 15.3,33.96 18.27,33.96 LD1.12
N$4
  Bottom 0.3: IC1.9 16.07,21.79 9.9,27.96 9.9,29.46 16.8,36.36 LD1.13
N$5
  Bottom 0.3: IC1.8 15.8,21.16 9.3,27.66 9.3,29.78 LD1.14
N$6
  Bottom 0.3: IC1.7 15.54,20.52 8.7,27.36 8.7,38.45 LD1.1
N$7
  Bottom 0.3: IC1.6 15.27,19.89 8.1,27.06 8.1,36.51 LD1.2
N$8
  Bottom 0.3: IC1.5 15.01,19.25 7.5,26.76 7.5,32.03 LD1.4
N$9
  Bottom 0.3: LD2.4 26.1,33.75 26.1,24.36 25.44,23.7 IC1.13
N$10
  Bottom 0.3: LD2.2 26.7,38.23 26.7,24.06 25.7,23.06 IC1.14
N$11
  Bottom 0.3: LD2.1 27.3,40.17 27.3,23.46 26.27,22.43 IC1.15
N$12
  Bottom 0.3: LD2.14 27.9,28.06 27.9,23.16 26.53,21.79 IC1.16
N$13
  Bottom 0.3: LD2.13 28.5,26.12 28.5,22.86 26.8,21.16 IC1.17
N$14
  Bottom 0.3: LD2.12 38.59,33.96 37.5,33.96 29.1,25.56 29.1,22.56 27.06,20.52 IC1.18
N$15
  Bottom 0.3: LD2.10 38.61,28.86 33.3,28.86 29.7,25.26 29.7,22.26 27.33,19.89 IC1.19
N$16
  Bottom 0.3: LD2.9 38.7,26.16 31.5,26.16 30.3,24.96 30.3,21.96 27.59,19.25 IC1.20
N$17
  Bottom 0.3: IC4.12 140.34,23.7 LD7.9
N$19
  Bottom 0.3: C16.+ 43.3,1.93 43,2.23 43,7 42.34,7.67 IC6.20 39.34,7.67 39,8 38.19,8 C9.1 38.05,7.3 37.75,7 19.27,7 X3.1
  Bottom 0.305: 43.28,1.76 C16.+
N$20
  Bottom 0.3: X3.2 18.32,5.45 D13.2 19.2,5.45 19.25,5.5 19.25,5.75 23,5.75 24.25,4.5 38.75,4.5 39.31,5.07 IC6.16
N$21
  Bottom 0.3: IC2.12 59.05,23.7 LD3.9
N$22
  Bottom 0.3: IC2.11 57.24,23.06 53.84,26.46 53.84,27.96 54.74,28.86 58.93,28.86 LD3.10
N$23
  Bottom 0.3: IC2.10 56.97,22.43 51.14,28.26 51.14,29.16 55.94,33.96 58.91,33.96 LD3.12
N$24
  Bottom 0.3: IC2.9 56.71,21.79 50.54,27.96 50.54,29.46 57.44,36.36 LD3.13
N$25
  Bottom 0.3: IC2.8 56.44,21.16 49.94,27.66 49.94,29.78 LD3.14
N$26
  Bottom 0.3: IC2.7 56.18,20.52 49.34,27.36 49.34,38.45 LD3.1
N$27
  Bottom 0.3: IC2.6 55.91,19.89 48.74,27.06 48.74,36.51 LD3.2
N$28
  Bottom 0.3: IC2.5 55.65,19.25 48.14,26.76 48.14,32.03 LD3.4
N$29
  Bottom 0.3: LD4.4 66.74,33.75 66.74,24.36 66.08,23.7 IC2.13
N$30
  Bottom 0.3: LD4.2 67.34,38.23 67.34,24.06 66.34,23.06 IC2.14
N$31
  Bottom 0.3: LD4.1 67.94,40.17 67.94,23.46 66.91,22.43 IC2.15
N$32
  Bottom 0.3: LD4.14 68.54,28.06 68.54,23.16 67.17,21.79 IC2.16
N$33
  Bottom 0.3: LD4.13 69.14,26.12 69.14,22.86 67.44,21.16 IC2.17
N$34
  Bottom 0.3: LD4.12 79.23,33.96 78.14,33.96 69.74,25.56 69.74,22.56 67.7,20.52 IC2.18
N$35
  Bottom 0.3: LD4.10 79.25,28.86 73.94,28.86 70.34,25.26 70.34,22.26 67.97,19.89 IC2.19
N$36
  Bottom 0.3: LD4.9 79.34,26.16 72.14,26.16 70.94,24.96 70.94,21.96 68.23,19.25 IC2.20
N$37
  Bottom 0.3: X3.3 18.22,3.55 D13.1 18.95,3.55 19.25,3.25 23.75,3.25 24.25,3.75 39,3.75 39.66,4.42 IC6.15
N$38
  Bottom 0.305: C21.1 83.63,5.32 | 83.63,5.32 83.54,5.24 83.54,3.98 Q1.1 | IC5.8 81.23,7.72 83.63,5.32
N$39
  Bottom 0.3: IC3.12 99.69,23.7 LD5.9
N$40
  Bottom 0.3: IC3.11 97.88,23.06 94.48,26.46 94.48,27.96 95.38,28.86 99.57,28.86 LD5.10
N$41
  Bottom 0.3: IC3.10 97.61,22.43 91.78,28.26 91.78,29.16 96.58,33.96 99.55,33.96 LD5.12
N$42
  Bottom 0.3: IC3.9 97.35,21.79 91.18,27.96 91.18,29.46 98.08,36.36 LD5.13
N$43
  Bottom 0.3: IC3.8 97.08,21.16 90.58,27.66 90.58,29.78 LD5.14
N$44
  Bottom 0.3: IC3.7 96.82,20.52 89.98,27.36 89.98,38.45 LD5.1
N$45
  Bottom 0.3: IC3.6 96.55,19.89 89.38,27.06 89.38,36.51 LD5.2
N$46
  Bottom 0.3: IC3.5 96.29,19.25 88.78,26.76 88.78,32.03 LD5.4
N$47
  Bottom 0.3: LD6.4 107.38,33.75 107.38,24.36 106.72,23.7 IC3.13
N$48
  Bottom 0.3: LD6.2 107.98,38.23 107.98,24.06 106.98,23.06 IC3.14
N$49
  Bottom 0.3: LD6.1 108.58,40.17 108.58,23.46 107.55,22.43 IC3.15
N$50
  Bottom 0.3: LD6.14 109.18,28.06 109.18,23.16 107.81,21.79 IC3.16
N$51
  Bottom 0.3: LD6.13 109.78,26.12 109.78,22.86 108.08,21.16 IC3.17
N$52
  Bottom 0.3: LD6.12 119.87,33.96 118.78,33.96 110.38,25.56 110.38,22.56 108.34,20.52 IC3.18
N$53
  Bottom 0.3: LD6.10 119.89,28.86 114.58,28.86 110.98,25.26 110.98,22.26 108.61,19.89 IC3.19
N$54
  Bottom 0.3: LD6.9 119.98,26.16 112.78,26.16 111.58,24.96 111.58,21.96 108.87,19.25 IC3.20
N$55
  Bottom 0.305: C19.2 88.12,7.27 87.86,7.52 86.34,7.52 86.08,7.78 86.08,8.24 Q1.3 86.08,8.33 86.08,9.55 85.8,9.84 IC5.7
N$57
  Bottom 0.3: IC4.11 138.52,23.06 135.12,26.46 135.12,27.96 136.02,28.86 140.21,28.86 LD7.10
N$58
  Bottom 0.3: IC4.10 138.25,22.43 132.42,28.26 132.42,29.16 137.22,33.96 140.19,33.96 LD7.12
N$59
  Bottom 0.3: IC4.9 137.99,21.79 131.82,27.96 131.82,29.46 138.72,36.36 LD7.13
N$60
  Bottom 0.3: IC4.8 137.72,21.16 131.22,27.66 131.22,29.78 LD7.14
N$61
  Bottom 0.3: IC4.7 137.46,20.52 130.62,27.36 130.62,38.45 LD7.1
N$62
  Bottom 0.3: IC4.6 137.19,19.89 130.02,27.06 130.02,36.51 LD7.2
N$63
  Bottom 0.3: IC4.5 136.93,19.25 129.42,26.76 129.42,32.03 LD7.4
N$64
  Bottom 0.3: LD8.4 148.02,33.75 148.02,24.36 147.36,23.7 IC4.13
N$65
  Bottom 0.3: LD8.2 148.62,38.23 148.62,24.06 147.62,23.06 IC4.14
N$66
  Bottom 0.3: LD8.1 149.22,40.17 149.22,23.46 148.19,22.43 IC4.15
N$67
  Bottom 0.3: LD8.14 149.82,28.06 149.82,23.16 148.45,21.79 IC4.16
N$68
  Bottom 0.3: LD8.13 150.42,26.12 150.42,22.86 148.72,21.16 IC4.17
N$69
  Bottom 0.3: LD8.12 160.51,33.96 159.42,33.96 151.02,25.56 151.02,22.56 148.98,20.52 IC4.18
N$70
  Bottom 0.3: LD8.10 160.53,28.86 155.22,28.86 151.62,25.26 151.62,22.26 149.25,19.89 IC4.19
N$71
  Bottom 0.3: LD8.9 160.62,26.16 153.42,26.16 152.22,24.96 152.22,21.96 149.51,19.25 IC4.20
N$72  (via drill 0.3)
  Top 0.3: v26.5,17.25 27,17.75 50.5,17.75 51,17.25 54.75,17.25 v55,17
  Bottom 0.3: IC1.22 25.77,17.98 v26.5,17.25 | IC2.2 55.35,17.35 v55,17
N$73  (via drill 0.3)
  Top 0.3: v68.25,17.25 68.75,17.75 70.5,17.75 70.75,18 79,18 79.25,17.75 80.75,17.75 81,18 92.5,18 93.25,17.25 93.75,17.25 94.5,18 95.75,18 v96.75,17
  Bottom 0.3: IC2.22 67.52,17.98 v68.25,17.25 | IC3.2 97.1,17.35 v96.75,17
N$74  (via drill 0.3)
  Top 0.3: v108.5,17.25 109,17.75 111.25,17.75 111.5,18 134.25,18 135,17.25 137.25,17.25 v137.5,17
  Bottom 0.3: IC3.22 107.77,17.98 v108.5,17.25 | IC4.2 137.85,17.35 v137.5,17
N$75  (via drill 0.3)
  Top 0.3: v149,17.25 149.75,18 150.5,18 150.75,17.75 152.25,17.75 152.5,18 169,18 169.75,17.25 170.5,17.25 172.75,17.25 v173,17
  Bottom 0.3: IC4.22 148.27,17.98 v149,17.25 | IC7.2 173.35,17.35 v173,17
N$76
  Bottom 0.3: IC1.23 25.15,17.35 26.75,15.75 26.75,14.85 R1.2
N$77
  Bottom 0.3: IC2.23 66.4,17.35 67.25,16.5 67.25,14.6 R5.2
N$78
  Bottom 0.3: IC3.23 106.65,17.35 108,16 108,14.6 R6.2
N$79
  Bottom 0.3: IC4.23 147.65,17.35 148.75,16.25 148.75,14.6 R7.2
N$80
  Bottom 0.3: IC7.23 182.9,17.35 183.5,16.75 183.5,14.4 R8.2
N$81  (via drill 0.3)
  Top 0.3: v105.25,9 v108,9
  Bottom 0.3: IC5.2 82.59,13.84 84,15.25 88.75,15.25 90.25,13.75 90.25,10.5 91.75,9 v105.25,9 | v108,9 111.5,9 112.41,9.9 IC10.14
N$82
  Bottom 0.3: IC5.10 78.94,3.06 80,2 111.5,2 113.67,4.17 IC10.2
N$85  (via drill 0.3)
  Top 0.3: v114.75,3.5 v111.75,3.5
  Bottom 0.3: IC10.4 111.14,4.12 v111.75,3.5 | IC9.4 117.3,5.55 115.25,3.5 v114.75,3.5
N$86
  Bottom 0.305: IC6.17 38.28,5.71 C11.2
N$88
  Bottom 0.3: IC7.12 175.76,24.76 177.25,26.25 180.92,26.25 LD9.9
N$89
  Bottom 0.3: IC7.11 173.94,23.06 173.7,23.3 173.7,23.9 177.3,27.5 179.74,27.5 LD9.10
N$90
  Bottom 0.3: LD9.12 180.83,33.96 177.86,33.96 173.06,29.16 173.06,23.04 173.67,22.43 IC7.10
N$91
  Bottom 0.3: LD9.13 179.36,36.36 172.46,29.46 172.46,22.44 173.11,21.79 IC7.9
N$92
  Bottom 0.3: LD9.14 171.86,29.78 171.86,21.84 172.54,21.16 IC7.8
N$93
  Bottom 0.3: LD9.1 171.26,38.45 171.26,21.54 172.28,20.52 IC7.7
N$94
  Bottom 0.3: LD9.2 170.66,36.51 170.66,21.24 172.01,19.89 IC7.6
N$95
  Bottom 0.3: LD9.4 170.06,32.03 170.06,20.94 171.75,19.25 IC7.5
RESET  (via drill 0.3)
  Top 0.3: X4.5 59.45,3.95 60.75,5.25 60.75,7.25 61.5,8 v65.5,8 | v84.25,14.25 v78.75,14.25
  Bottom 0.3: v65.5,8 68,8 69.25,9.25 69.25,13.25 74.75,18.75 76.5,18.75 77.34,17.91 IC5.29 77.34,15.16 78.25,14.25 v78.75,14.25 | R4.2 C13.1 84.4,14.1 v84.25,14.25
RXD  (via drill 0.3)
  Top 0.3: v77.5,22 76.5,21 70.75,21 70.5,21.25 69,21.25 68.75,21 54,21 53.5,21.5 52.75,21.5 52.25,21 50.5,21 v49,22.5
  Bottom 0.3: IC5.30 78.14,21.36 v77.5,22 | IC6.1 49.37,12.87 49.5,13 49.5,22 v49,22.5
SCK  (via drill 0.3)
  Top 0.3: v65.5,5.25 63.35,5.25 X4.3 | v13.5,18.25 14.75,19.5 27.75,19.5 28.75,18.5 29.75,18.5 30,18.75 50.75,18.75 v51.25,18.25 v54,18.25 54.5,18.75 68.75,18.75 69,18.5 70.25,18.5 70.5,18.75 79.25,18.75 79.5,18.5 80.5,18.5 80.75,18.75 93,18.75 v93.5,18.25 94,18.75 109.75,18.75 110,18.5 111,18.5 111.25,18.75 134.75,18.75 v135.25,18.25 135.75,18.75 150.75,18.75 151,18.5 152,18.5 152.25,18.75 169.5,18.75 v170,18.25
  Bottom 0.3: IC5.17 72.65,5.9 71.5,4.75 66,4.75 v65.5,5.25 | IC1.3 13.77,17.98 v13.5,18.25 | IC7.3 170.27,17.98 v170,18.25 | IC4.3 135.52,17.98 v135.25,18.25 | IC3.3 93.77,17.98 v93.5,18.25 | IC2.3 54.27,17.98 v54,18.25 | X4.3 61.99,3.74 60.75,2.5 58.5,2.5 51.25,9.75 v51.25,18.25
SYNC  (via drill 0.3)
  Top 0.3: v113.5,2.5 111,2.5 v109.75,3.75
  Bottom 0.3: IC10.5 109.86,3.87 v109.75,3.75 109,3 104.82,3 102.82,5 101.32,5 JP1.1 101.24,7.61 R2.2 | IC9.2 118.25,2.75 118,2.5 v113.5,2.5
TXD  (via drill 0.3)
  Top 0.3: v49,23.75 51,21.75 52,21.75 52.5,22.25 53.75,22.25 54.25,21.75 68.5,21.75 68.75,22 70.75,22 71,21.75 75.75,21.75 77,23 77.75,23 v78.75,22
  Bottom 0.3: v49,23.75 50.25,22.5 50.25,10.75 49.77,10.27 IC6.5 | IC5.31 78.94,21.81 v78.75,22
